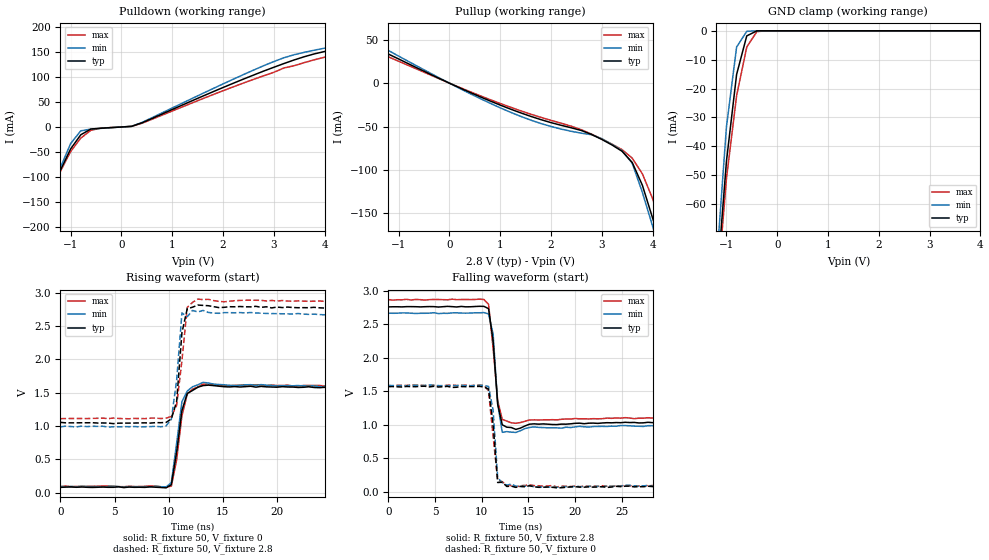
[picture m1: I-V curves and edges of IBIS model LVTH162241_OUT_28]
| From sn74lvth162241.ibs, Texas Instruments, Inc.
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|  Model LVTH162241 Output_28
[Model]   LVTH162241_OUT_28
Model_type  3-state
Polarity   Non-Inverting
Enable   Active-Low
Vmeas = 1.5V
Cref = 50pF
Rref = 500
Vref = 0
| variable   typ   min   max
C_comp   9pf   NA   NA
[Temperature Range]   40   -25   100
| Ambient temperature   25   -40   85
[Voltage range]   2.8   2.7   2.9
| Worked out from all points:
|   slope of the pulldown table from 0 to 0.42 V, typ, clamps not added: 46.8 ohm
|   slope of the pullup table from 0 to 0.42 V, typ, clamps not added: 38.1 ohm
|   GND clamp passes 1 mA (typ) near -0.51 V on its own axis
|   rising waveform, R_fixture 50, V_fixture 0: 20-80 % time 793ps typ, 721ps min, 824ps max; typ from 0.078 V to 1.56 V
|   falling waveform, R_fixture 50, V_fixture 2.8: 20-80 % time 619ps typ, 476ps min, 706ps max; typ from 2.76 V to 1.04 V
|   rising waveform, R_fixture 50, V_fixture 2.8: 20-80 % time 506ps typ, 616ps min, 708ps max; typ from 1.05 V to 2.77 V
|   falling waveform, R_fixture 50, V_fixture 0: 20-80 % time 600ps typ, 505ps min, 661ps max; typ from 1.57 V to 0.085 V
[Pullup]
|   Voltage   I(typ)   I(min)   I(max)
-5V       77.96uA    75.56uA    77.6uA
-2.4V     66.8uA     62.42uA    67.53uA
-2.2V     66.8uA     54.14mA    67.12uA
-2V       66.8uA     62.57mA    66.73uA
-1.8V     50.1mA     56.46mA    66.36uA
-1.6V     44.54mA    50.55mA    65.98uA
-1.4V     38.94mA    43.28mA    35.4mA
2.8V      -59.19mA   -59.43mA   -58.78mA
3.6V      -91.39mA   -92.25mA   -86.41mA
4V        -155.2mA   -164.5mA   -132.8mA
4.2V      -192.7mA   -203.2mA   -171.3mA
10V       -1.282A    -1.326A    -1.286A
[Pulldown]
|   Voltage   I(typ)   I(min)   I(max)
-5V       -1.373A    -1.496A    -1.193A
-1.6V     -216.7mA   -223mA     -202.4mA
-1.4V     -148.7mA   -148.1mA   -144.2mA
-1.2V     -86.4mA    -80.74mA   -88.45mA
-1V       -43.99mA   -33.37mA   -49.29mA
-800mV    -15.66mA   -7.804mA   -22.3mA
-600mV    -4.186mA   -4.185mA   -6.717mA
200mV     1.16mA     1.253mA    1.073mA
3.4V      133.7mA    144.2mA    122.2mA
4.6V      162.1mA    168.1mA    151mA
6.8V      191.2mA    198.9mA    178.8mA
10V       221.9mA    200mA      208.2mA
[GND Clamp]
|   Voltage   I(typ)   I(min)   I(max)
-5V       -1.546A    -1.736A    -1.341A
-1.2V     -90.16mA   -82.13mA   -93.95mA
-1V       -45.24mA   -33.32mA   -51.26mA
-800mV    -15.13mA   -5.621mA   -22.5mA
-600mV    -1.753mA   -176.9uA   -5.607mA
-400mV    -7.631uA   -72.38nA   -259.8uA
-200mV    -5.356nA   -23.89nA   -733.2nA
5V        42.74nA    331nA      79.76nA
[Ramp]
| variable   typ   min   max
dV/dt_r   1.165E-00/7.550E-10  1.146E-00/6.510E-10  1.188E-00/7.450E-10
dV/dt_f   1.440E+00/5.540E-10  1.378E+00/4.780E-10  1.500E+00/6.310E-10
R_load = 50
[Rising Waveform]
R_fixture = 50
V_fixture = 0
V_fixture_min = 0
V_fixture_max = 0
C_fixture = 0
L_fixture = 0
|   Time   V(typ)   V(min)   V(max)
0s        78.13mV    94mV       89.27mV
9.766ns   70.95mV    83.47mV    82.86mV
10.25ns   117.8mV    149.2mV    96.28mV
10.74ns   605.9mV    739mV      489.7mV
11.23ns   1.23V      1.363V     1.152V
11.72ns   1.488V     1.523V     1.477V
13.18ns   1.606V     1.655V     1.629V
16.11ns   1.591V     1.607V     1.609V
31.25ns   1.557V     1.573V     1.59V
49.71ns   1.565V     1.591V     1.591V
[Falling Waveform]
R_fixture = 50
V_fixture = 2.8
V_fixture_min = 2.7
V_fixture_max = 2.9
C_fixture = 0
L_fixture = 0
|   Time   V(typ)   V(min)   V(max)
0s        2.76V      2.667V     2.868V
9.766ns   2.769V     2.672V     2.876V
10.74ns   2.734V     2.655V     2.798V
11.23ns   2.251V     2.355V     2.147V
11.72ns   1.31V      1.318V     1.364V
12.21ns   1.002V     889.4mV    1.082V
13.18ns   960.9mV    891.3mV    1.032V
13.67ns   933.2mV    888.2mV    1.024V
15.63ns   1.016V     970.8mV    1.075V
49.71ns   1.04V      987.7mV    1.112V
[Rising Waveform]
R_fixture = 50
V_fixture = 2.8
V_fixture_min = 2.7
V_fixture_max = 2.9
C_fixture = 0
L_fixture = 0
|   Time   V(typ)   V(min)   V(max)
0s        1.054V     987.1mV    1.11V
9.277ns   1.049V     987.9mV    1.112V
10.25ns   1.106V     1.1V       1.144V
10.74ns   1.365V     1.682V     1.308V
11.23ns   2.4V       2.697V     1.979V
11.72ns   2.759V     2.639V     2.779V
12.21ns   2.783V     2.734V     2.855V
12.7ns    2.815V     2.712V     2.904V
31.25ns   2.75V      2.647V     2.844V
49.71ns   2.765V     2.67V      2.871V
[Falling Waveform]
R_fixture = 50
V_fixture = 0
V_fixture_min = 0
V_fixture_max = 0
C_fixture = 0
L_fixture = 0
|   Time   V(typ)   V(min)   V(max)
0s        1.571V     1.589V     1.586V
9.766ns   1.575V     1.591V     1.594V
10.25ns   1.566V     1.59V      1.589V
10.74ns   1.535V     1.574V     1.51V
11.23ns   1.012V     1.216V     830.2mV
11.72ns   141.1mV    214.8mV    175.6mV
12.21ns   145.4mV    137.3mV    153.4mV
12.7ns    81.94mV    101.5mV    100.7mV
18.07ns   61.19mV    70.65mV    74.01mV
49.71ns   85.3mV     88.81mV    86.52mV
